{attribute 'pack_mode' := '1'}
TYPE SerialComData :
STRUCT
	FrameHeader	: BYTE;
	Data1		: LREAL;
	Data2		: LREAL;
	Data3		: LREAL;
	Data4		: LREAL;
	Data5		: LREAL;
	CRC			: WORD;
	FrameEnd	: BYTE;
END_STRUCT
END_TYPE
